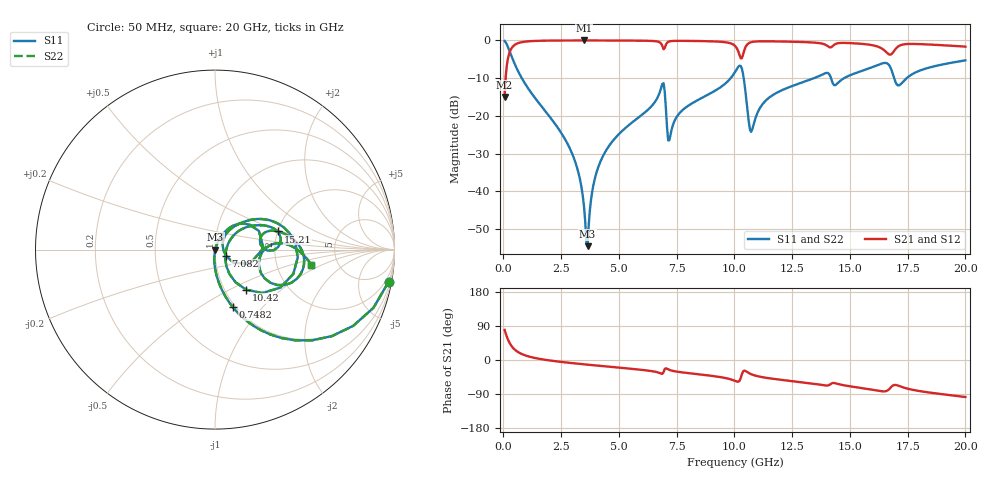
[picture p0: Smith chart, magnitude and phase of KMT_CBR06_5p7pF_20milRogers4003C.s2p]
! Data measured by Modelithics Inc. support@modelithics.com 813-866-6335
! KEMET CBR0603 5.7pF, Pad Width= 0.851mm, Pad Length= 0.64mm, Pad Gap= 0.62mm, 20mil Rogers 4003C substrate Data, January 2022
# hz S ma R 50
! 2 Port Network Data from SP1.SP block
! freq  magS11  angS11  magS21  angS21  magS12  angS12  magS22  angS22
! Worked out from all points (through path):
!   401 points, 50 MHz to 20 GHz, reference 50 ohm
!   highest |S21| = -0.02 dB at 3.491 GHz (marker M1); lowest = -15.0 dB at 50 MHz (marker M2)
!   group delay of S21, straight-line fit = 15.1 ps
!   lowest |S11| = -54.6 dB at 3.641 GHz (marker M3), VSWR 1.00, Z = 50.2 + j0.0525 ohm
!   |S11| at or under -10 dB: 792.3 MHz to 9.84 GHz (9.047 GHz wide, 170 % of centre); 10.4 GHz to 13.46 GHz (3.056 GHz wide, 25.6 % of centre); 14.18 GHz to 14.75 GHz (572.9 MHz wide, 3.96 % of centre)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
!   |S22| runs from -54.6 to -0.1 dB; largest |S21 - S12| = 0
!   S11 on the Smith chart (normalised r, x): 50 MHz: 1, -11; 748.2 MHz: 0.97, -0.70; 7.082 GHz: 1.13, -0.08; 10.42 GHz: 1.26, -0.61; 15.21 GHz: 2.01, +0.47; 20 GHz: 3.18, -0.76
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5e7  0.984 -10.4  0.1777 79.6  0.1777 79.6  0.984 -10.4
2.99375e8  0.6763 -48.4  0.736 41.5  0.736 41.5  0.6763 -48.4
7.4825e8  0.3343 -72.9  0.9416 17.0  0.9416 17.0  0.3343 -72.9
2.74325e9  0.04437 -94.9  0.9975 -6.7  0.9975 -6.7  0.04437 -94.9
3.391625e9  0.01066 -92.3  0.9982 -10.8  0.9982 -10.8  0.01066 -92.3
3.491375e9  0.006102 -86.2  0.9983 -11.4  0.9983 -11.4  0.006102 -86.2
3.641e9  0.001867 16.3  0.9982 -12.3  0.9982 -12.3  0.001867 16.3
3.94025e9  0.01401 68.9  0.998 -14.1  0.998 -14.1  0.01401 68.9
4.33925e9  0.03051 70.2  0.9975 -16.4  0.9975 -16.4  0.03051 70.2
6.73325e9  0.1926 47.8  0.9526 -33.6  0.9526 -33.6  0.1926 47.8
6.93275e9  0.2704 1.8  0.7635 -31.9  0.7635 -31.9  0.2704 1.8
7.082375e9  0.0706 -29.6  0.9296 -23.3  0.9296 -23.3  0.0706 -29.6
7.232e9  0.05616 39.4  0.9761 -27.2  0.9761 -27.2  0.05616 39.4
1.0025e10  0.38 22.4  0.8465 -55.2  0.8465 -55.2  0.38 22.4
1.0424e10  0.2832 -52.1  0.7344 -28.0  0.7344 -28.0  0.2832 -52.1
1.072325e10  0.06127 -7.5  0.946 -37.4  0.946 -37.4  0.06127 -7.5
1.147138e10  0.1712 38.1  0.9728 -47.9  0.9728 -47.9  0.1712 38.1
1.336662e10  0.3087 25.7  0.9389 -62.1  0.9389 -62.1  0.3087 25.7
1.5212e10  0.3652 16.1  0.914 -71.3  0.914 -71.3  0.3652 16.1
1.670825e10  0.4642 -23.4  0.6486 -76.4  0.6486 -76.4  0.4642 -23.4
1.710725e10  0.2527 -11.5  0.8376 -68.0  0.8376 -68.0  0.2527 -11.5
2e10  0.5434 -8.9  0.8266 -97.7  0.8266 -97.7  0.5434 -8.9
